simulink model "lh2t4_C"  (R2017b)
settings: Solver=ode45  StartTime=0.0  StopTime=10  RelTol=1e-3  EnableMultiTasking=on
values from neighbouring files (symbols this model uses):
  m0 = 1000    [lh2t4_DOC.m]
libraries: mat24129_lib x3

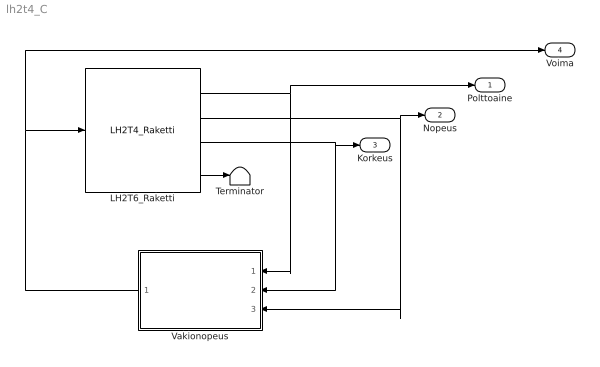
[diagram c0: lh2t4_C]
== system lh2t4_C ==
  LH2T6_Raketti : mat24129_lib/LH2T4_Raketti
  Terminator : Terminator
  Vakionopeus : Subsystem
  Polttoaine : Outport
  Nopeus : Outport  Port=2
  Korkeus : Outport  Port=3
  Voima : Outport  Port=4
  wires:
  LH2T6_Raketti/1 -> Polttoaine/1, Vakionopeus/1(Polttoaine)
  LH2T6_Raketti/2 -> Nopeus/1, Vakionopeus/3(Nopeus)
  LH2T6_Raketti/3 -> Korkeus/1, Vakionopeus/2(Korkeus)
  Vakionopeus/1(Voima) -> Voima/1, LH2T6_Raketti/1
  LH2T6_Raketti/4 -> Terminator/1

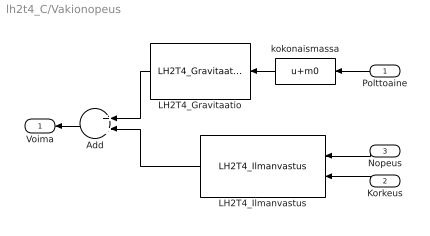
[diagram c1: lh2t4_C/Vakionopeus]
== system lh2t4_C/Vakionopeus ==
  Polttoaine : Inport
  Korkeus : Inport  Port=2
  Nopeus : Inport  Port=3
  Add : Sum
  LH2T4_Gravitaatio : mat24129_lib/LH2T4_Gravitaatio
  LH2T4_Ilmanvastus : mat24129_lib/LH2T4_Ilmanvastus
  kokonaismassa : Fcn  Expr=u+m0
  Voima : Outport
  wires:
  LH2T4_Ilmanvastus/1 -> Add/2
  Polttoaine/1 -> kokonaismassa/1
  Add/1 -> Voima/1
  LH2T4_Gravitaatio/1 -> Add/1
  kokonaismassa/1 -> LH2T4_Gravitaatio/1
  Korkeus/1 -> LH2T4_Ilmanvastus/2
  Nopeus/1 -> LH2T4_Ilmanvastus/1
